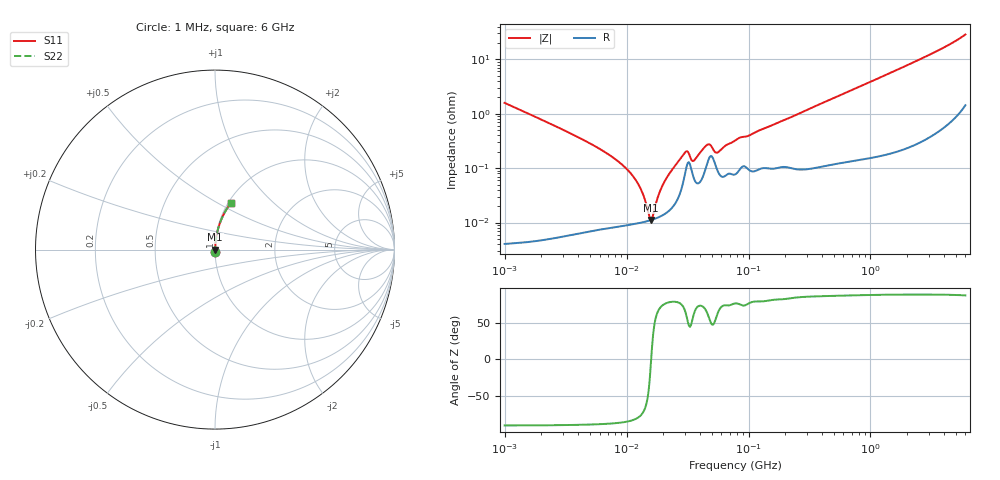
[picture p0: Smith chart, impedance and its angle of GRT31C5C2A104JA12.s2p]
!Murata Part Number: GRT31C5C2A104JA12
!These Parameters are Measured in Series Mode Connection
!Data Generated on Jun 19, 2026
!  o--ll--o
!Port1  Port2
!  o------o
!Operation Temp=25[degC], DC Bias Voltage=0[V]
!Freq. Start=1000[kHz] Stop=6[GHz] 401[Steps]
# Hz S RI R 50
!Freq.(Hz) S11(Real) S11(Imag) S21(Real) S21(Imag) S12(Real) S12(Imag) S22(Real) S22(Imag)
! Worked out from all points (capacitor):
!   401 points, 1 MHz to 6 GHz, reference 50 ohm
!   read as one part in series: C = 100 nF near 1.044 MHz
!   lowest |Z| = 11.1 mohm at 15.83 MHz (marker M1)
!   series resonance near 15.91 MHz, so ESL is about 1 nH
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1000000  0.000291 -0.0158  0.9997 0.0158  0.9997 0.0158  0.000291 -0.0158
4293785  7.61e-05 -0.00342  0.9999 0.00342  0.9999 0.00342  7.61e-05 -0.00342
7395623  8.26e-05 -0.00169  0.9999 0.00169  0.9999 0.00169  8.26e-05 -0.00169
1.047372e7  9.11e-05 -0.000867  0.9999 0.000867  0.9999 0.000867  9.11e-05 -0.000867
1.301831e7  9.92e-05 -0.000411  0.9999 0.000411  0.9999 0.000411  9.92e-05 -0.000411
1.389603e7  0.000102 -0.000278  0.9999 0.000278  0.9999 0.000278  0.000102 -0.000278
1.515906e7  0.000108 -9.97e-05  0.9999 9.97e-05  0.9999 9.97e-05  0.000108 -9.97e-05
1.583299e7  0.000111 -1.01e-05  0.9999 1.01e-05  0.9999 1.01e-05  0.000111 -1.01e-05
1.653689e7  0.000114 8.02e-05  0.9999 -8.02e-05  0.9999 -8.02e-05  0.000114 8.02e-05
1.843659e7  0.000126 0.000312  0.9999 -0.000312  0.9999 -0.000312  0.000126 0.000312
2.194036e7  0.00016 0.000719  0.9998 -0.000719  0.9998 -0.000719  0.00016 0.000719
3.040356e7  0.000864 0.00179  0.9991 -0.00179  0.9991 -0.00179  0.000864 0.00179
3.175522e7  0.00125 0.00158  0.9987 -0.00158  0.9987 -0.00158  0.00125 0.00158
3.540316e7  0.000676 0.00118  0.9993 -0.00118  0.9993 -0.00118  0.000676 0.00118
4.596069e7  0.00124 0.0024  0.9988 -0.0024  0.9988 -0.0024  0.00124 0.0024
4.800399e7  0.0016 0.00221  0.9984 -0.00221  0.9984 -0.00221  0.0016 0.00221
5.589783e7  0.000885 0.00173  0.9991 -0.00173  0.9991 -0.00173  0.000885 0.00173
7.745967e7  0.000775 0.00312  0.9992 -0.00312  0.9992 -0.00312  0.000775 0.00312
3.325952e8  0.00115 0.0129  0.9988 -0.0129  0.9988 -0.0129  0.00115 0.0129
1.428092e9  0.00486 0.055  0.9951 -0.055  0.9951 -0.055  0.00486 0.055
3.335232e9  0.0217 0.1309  0.9783 -0.1309  0.9783 -0.1309  0.0217 0.1309
6e9  0.0871 0.258  0.9129 -0.258  0.9129 -0.258  0.0871 0.258
